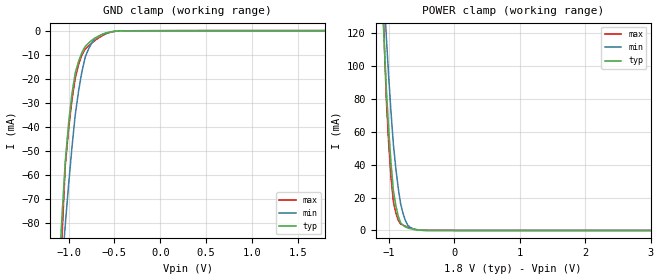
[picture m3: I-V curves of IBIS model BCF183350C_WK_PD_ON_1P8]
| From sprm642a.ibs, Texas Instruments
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|   Model Cell BCF183350C_WK_PD_ON_1P8
|BCF183350C_WK_PD_ON_1P8
[Model]   BCF183350C_WK_PD_ON_1P8
Model_type   Input
Polarity   Non-Inverting
Vinl =  0.63
Vinh =  1.17
C_comp   1.111906p   0.9691991p   1.265789p
[Model Spec]
Vinl   0.63   0.63   0.63
Vinh   1.17   1.17   1.17
[Temperature Range]   25   155   -40
[Voltage Range]   1.8   1.62   1.98
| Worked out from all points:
|   GND clamp passes 1 mA (typ) near -0.59 V on its own axis
|   POWER clamp passes 1 mA (typ) near -0.66 V on its own axis
| Nom Voltages:
|   VDD=1.2, VDDS=1.8, VSS=0
| Min Voltages:
|   VDD=1.08, VDDS=1.62, VSS=0
| Max Voltages:
|   VDD=1.32, VDDS=1.98, VSS=0
[POWER_clamp]
|   voltage   I(typ)   I(min)   I(max)
-1.8V     884.3mA    853.3mA    1.248A
-1.109V   150.5mA    176mA      165.6mA
-1.073V   117.6mA    146.3mA    120.4mA
-1.036V   86.45mA    117.9mA    79.86mA
-1V       61.3mA     93.4mA     52.74mA
-963.6mV  40.45mA    71.37mA    31.85mA
-927.3mV  23.88mA    51.84mA    17.18mA
-818.2mV  4.712mA    16.29mA    3.969mA
-745.5mV  2.166mA    6.116mA    2.588mA
-636.4mV  820.5uA    1.141mA    1.102mA
-454.5mV  62.76uA    84.47uA    90.44uA
3.6V      0A         0A         0A
[GND_clamp]
|   voltage   I(typ)   I(min)   I(max)
-1.8V     -722.8mA   -541.3mA   -1.24A
-1.109V   -103.2mA   -119.1mA   -124.9mA
-1.073V   -77.6mA    -99.56mA   -86.65mA
-1.036V   -54.4mA    -80.72mA   -56.17mA
-1V       -38.53mA   -63.93mA   -40.95mA
-963.6mV  -26.24mA   -48.65mA   -28.78mA
-927.3mV  -17.51mA   -34.88mA   -19.66mA
-890.9mV  -12.74mA   -24.97mA   -14.04mA
-818.2mV  -6.487mA   -10.88mA   -7.582mA
-709.1mV  -2.982mA   -3.215mA   -3.97mA
-418.2mV  -55.59uA   -81.47uA   -71.73uA
1.8V      28.03uA    11.74uA    55.46uA
